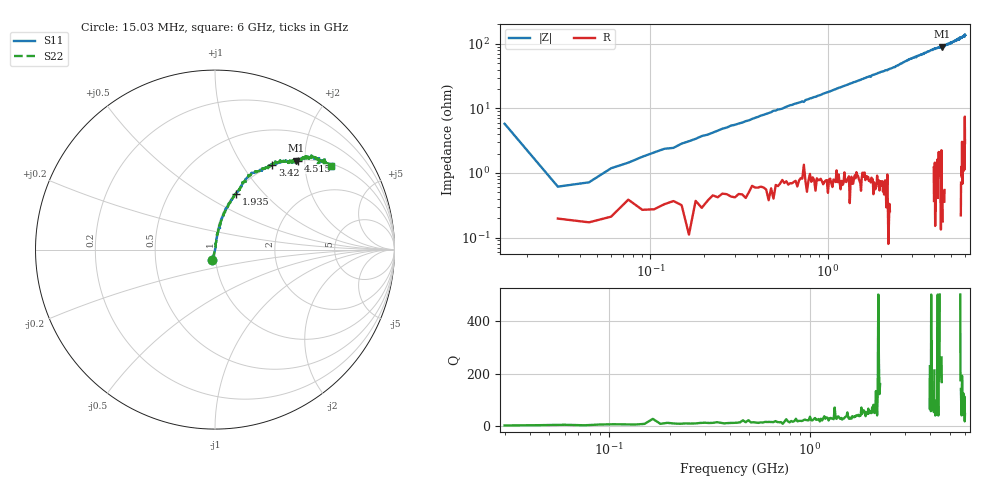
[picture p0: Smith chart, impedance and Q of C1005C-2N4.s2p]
!	Network	Analyzer	HP8753E.07.74:	Oct	30	2002	Serial	No.	JP38451487
!	Hewlett-Packard
!	7	Sep	2009	8:19:55
!	Frequency	S11	S21	S12	S22
#	HZ	S	RI	R	50
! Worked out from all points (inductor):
!   400 points, 15.03 MHz to 6 GHz, reference 50 ohm
!   read as one part in series: L = 2.95 nH near 45.03 MHz
!   highest Q = 200 at 4.41 GHz (marker M1), where L = 3.26 nH
!   S11 on the Smith chart (normalised r, x): 15.03 MHz: 0.97, -0.11; 1.935 GHz: 1.01, +0.71; 3.42 GHz: 0.98, +1.38; 4.515 GHz: 1.01, +1.86; 6 GHz: 1.07, +2.73
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1.502992e7  -0.014 -0.0574  1.01 0.0574  1.01 0.0574  -0.014 -0.0574
3.002985e7  0.00199 0.00579  0.998 -0.00579  0.998 -0.00579  0.00199 0.00579
4.502978e7  0.00153 0.00693  0.998 -0.00693  0.998 -0.00693  0.00153 0.00693
6.00297e7  0.00247 0.0116  0.998 -0.0116  0.998 -0.0116  0.00247 0.0116
1.050295e8  0.00331 0.0205  0.997 -0.0205  0.997 -0.0205  0.00331 0.0205
1.95029e8  0.00448 0.0369  0.996 -0.0369  0.996 -0.0369  0.00448 0.0369
2.850286e8  0.00731 0.0533  0.993 -0.0533  0.993 -0.0533  0.00731 0.0533
4.950275e8  0.0125 0.0903  0.988 -0.0903  0.988 -0.0903  0.0125 0.0903
7.350263e8  0.0281 0.12  0.972 -0.12  0.972 -0.12  0.0281 0.12
7.650262e8  0.0234 0.133  0.977 -0.133  0.977 -0.133  0.0234 0.133
1.020025e9  0.0391 0.173  0.961 -0.173  0.961 -0.173  0.0391 0.173
1.335023e9  0.0582 0.227  0.942 -0.227  0.942 -0.227  0.0582 0.227
1.93502e9  0.117 0.312  0.883 -0.312  0.883 -0.312  0.117 0.312
2.01002e9  0.124 0.32  0.876 -0.32  0.876 -0.32  0.124 0.32
2.415018e9  0.154 0.375  0.846 -0.375  0.846 -0.375  0.154 0.375
3.015015e9  0.263 0.452  0.737 -0.452  0.737 -0.452  0.263 0.452
3.420013e9  0.32 0.474  0.68 -0.474  0.68 -0.474  0.32 0.474
4.00501e9  0.417 0.496  0.583 -0.496  0.583 -0.496  0.417 0.496
4.410008e9  0.45 0.495  0.55 -0.495  0.55 -0.495  0.45 0.495
4.515007e9  0.464 0.496  0.536 -0.496  0.536 -0.496  0.464 0.496
5.010005e9  0.519 0.513  0.481 -0.513  0.481 -0.513  0.519 0.513
6e9  0.647 0.466  0.353 -0.466  0.353 -0.466  0.647 0.466
